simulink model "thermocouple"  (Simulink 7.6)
settings: Solver=ode14x  StartTime=0.0  StopTime=N  RelTol=1e-3
InitFcn:
  | close all
  | clear all
  | clc
  | N=10;
  | fem_temp_thermocouple
StopFcn:
  | close all
  | load temp.mat
  | plotyy(x(1,:),x(2,:),x(1,:),x(3,:))
  | title('Température d''entrée et f.e.m du thermocouple')
  | xlabel('temps')
  | grid
  | 
  | delete *.mat
undefined symbols (not defined in the file or in its folder): c0, c1, c2, c3, c4, c5, c6, c7, c8, c9
libraries: fl_lib x7, nesl_utility x4, elec_lib x1

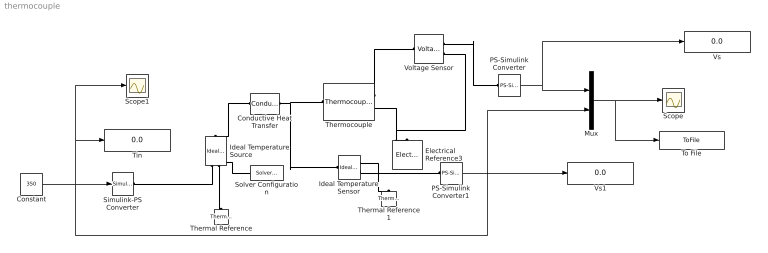
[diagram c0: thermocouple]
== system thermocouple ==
  Conductive Heat Transfer : fl_lib/Thermal/Thermal Elements/Conductive Heat Transfer  DialogController=NetworkEngine.DynNeDlgSource  SystemSampleTime=-1  area=1e-02 m^2  thickness=0.1 m  th_cond=401 W/(m*K)  Q_Log=off  T_Log=off  LocalVarNames=|Q|T  LocalVarDescs=|Q|T  LocalVarLogging=[0 0]
  Constant : Constant  Value=350
  Electrical Reference3 : fl_lib/Electrical/Electrical Elements/Electrical Reference  DialogController=NetworkEngine.DynNeDlgSource  SystemSampleTime=-1  i_Log=off  LocalVarNames=|i  LocalVarDescs=|i  LocalVarLogging=0
  Ideal Temperature Sensor : fl_lib/Thermal/Thermal Sensors/Ideal Temperature Sensor  DialogController=NetworkEngine.DynNeDlgSource  SystemSampleTime=-1  Qs_Log=off  Ts_Log=off  LocalVarNames=|Qs|Ts  LocalVarDescs=|Qs|Ts  LocalVarLogging=[0 0]
  Ideal Temperature Source : fl_lib/Thermal/Thermal Sources/Ideal Temperature Source  DialogController=NetworkEngine.DynNeDlgSource  SystemSampleTime=-1  Q_Log=off  T_Log=off  LocalVarNames=|Q|T  LocalVarDescs=|Q|T  LocalVarLogging=[0 0]
  Mux : Mux  Inputs=2
  PS-Simulink Converter : nesl_utility/PS-Simulink Converter  DialogController=NetworkEngine.DynNeUtilDlgSource  SystemSampleTime=-1  PhysicalDomain=network_engine_domain  LeftPortType=input  RightPortType=output  SubClassName=ps_output  Unit=1  AffineConversion=off
  PS-Simulink Converter1 : nesl_utility/PS-Simulink Converter  DialogController=NetworkEngine.DynNeUtilDlgSource  SystemSampleTime=-1  PhysicalDomain=network_engine_domain  LeftPortType=input  RightPortType=output  SubClassName=ps_output  Unit=1  AffineConversion=off
  Scope : Scope
  Scope1 : Scope
  Simulink-PS Converter : nesl_utility/Simulink-PS Converter  DialogController=NetworkEngine.DynNeUtilDlgSource  SystemSampleTime=-1  PhysicalDomain=network_engine_domain  LeftPortType=input  RightPortType=output  SubClassName=ps_input  Unit=1  AffineConversion=off  InputFilterTimeConstant=.001  UdotUserProvided=0
  Solver Configuration : nesl_utility/Solver Configuration  DialogController=NetworkEngine.DynNeUtilDlgSource  SystemSampleTime=-1  PhysicalDomain=network_engine_domain  LeftPortType=input  RightPortType=generic  SubClassName=solver  Accelerate=off  Profile=off  ResidualTolerance=1e-9  MaxNonlinIter=12  MaxModeIter=2  DoFixedCost=off  UseLocalSampling=off  DoDC=on  LinearAlgebra=Full  LocalSolverSampleTime=.001  LocalSolverChoice=NE_BACKWARD_EULER_ADVANCER  UseLocalSolver=off
  Thermal Reference : fl_lib/Thermal/Thermal Elements/Thermal Reference  DialogController=NetworkEngine.DynNeDlgSource  SystemSampleTime=-1  Q_Log=off  LocalVarNames=|Q  LocalVarDescs=|Q  LocalVarLogging=0
  Thermal Reference1 : fl_lib/Thermal/Thermal Elements/Thermal Reference  DialogController=NetworkEngine.DynNeDlgSource  SystemSampleTime=-1  Q_Log=off  LocalVarNames=|Q  LocalVarDescs=|Q  LocalVarLogging=0
  Thermocouple : elec_lib/Sensors/Thermocouple  DialogController=NetworkEngine.DynNeDlgSource  SystemSampleTime=-1  Cvec=[ c0 c1 c2 c3 c4 c5 c6 c7 c8 c9 ]  T0=0 C  tc=1 s  K_d=0.001 W/K  init_temp=25 C  LocalVarLogging=[]
  Tin : Display
  To File : ToFile  Filename=temp.mat  MatrixName=x
  Voltage Sensor : fl_lib/Electrical/Electrical Sensors/Voltage Sensor  DialogController=NetworkEngine.DynNeDlgSource  SystemSampleTime=-1  i1_Log=off  v1_Log=off  LocalVarNames=|i1|v1  LocalVarDescs=|i1|v1  LocalVarLogging=[0 0]
  Vs : Display
  Vs1 : Display
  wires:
  PS-Simulink Converter/1 -> Mux/1, Vs/1
  Mux/1 -> To File/1, Scope/1
  Constant/1 -> Simulink-PS Converter/1, Mux/2, Tin/1, Scope1/1
  PS-Simulink Converter1/1 -> Vs1/1
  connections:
  Ideal Temperature Source/RConn2 -- Thermal Reference/LConn1 -- Solver Configuration/RConn1
  Conductive Heat Transfer/RConn1 -- Thermocouple/RConn1 -- Ideal Temperature Sensor/LConn1
  Voltage Sensor/RConn2 -- Thermocouple/LConn2 -- Electrical Reference3/LConn1
  Thermocouple/LConn1 -- Voltage Sensor/LConn1
  Ideal Temperature Source/RConn1 -- Simulink-PS Converter/RConn1
  Conductive Heat Transfer/LConn1 -- Ideal Temperature Source/LConn1
  Ideal Temperature Sensor/RConn1 -- Thermal Reference1/LConn1
  Ideal Temperature Sensor/RConn2 -- PS-Simulink Converter1/LConn1
  PS-Simulink Converter/LConn1 -- Voltage Sensor/RConn1
